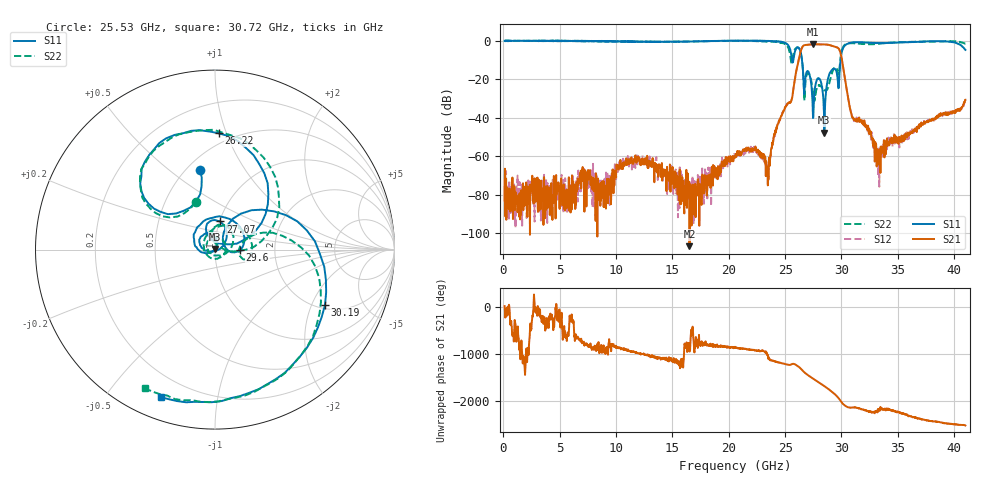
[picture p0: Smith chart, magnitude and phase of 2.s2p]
!The following data was pulled from an Agilent PNA
!This sNp file was generated from the data in the RF Test software
!NOTE:  Smoothing/Math/Corrections applied on any given trace ARE included in the data saved here
# MHz S dB R 50
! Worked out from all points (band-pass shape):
!   1601 points, 100 MHz to 41 GHz, reference 50 ohm
!   highest |S21| = -1.73 dB at 27.48 GHz (marker M1); lowest = -106.6 dB at 16.51 GHz (marker M2)
!   |S21| within 3 dB of the highest: 26.42 GHz to 29.82 GHz (3.401 GHz wide, 12.1 % of centre)
!   lowest |S11| = -47.7 dB at 28.47 GHz (marker M3), VSWR 1.01, Z = 50 + j0.411 ohm
!   |S11| at or under -10 dB: 25.61358 GHz to 25.72955 GHz (116 MHz wide, 0.452 % of centre); 26.5 GHz to 29.92 GHz (3.42 GHz wide, 12.1 % of centre)
!   |S22| runs from -31.2 to 0.2 dB; largest |S21 - S12| = 0.0062
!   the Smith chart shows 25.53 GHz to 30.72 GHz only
!   S11 on the Smith chart (normalised r, x): 25.53 GHz: 0.58, +0.65; 26.22 GHz: 0.42, +0.94; 27.07 GHz: 1.01, +0.32; 29.6 GHz: 1.32, -0.00; 30.19 GHz: 2.17, -2.52; 30.72 GHz: 0.10, -0.70
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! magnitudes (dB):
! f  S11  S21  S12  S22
! 100 MHz  0.0  -82.9  -75.6  0.0
! 6.925 GHz  -0.1  -68.3  -71.2  -0.2
! 8.536 GHz  -0.3  -76.6  -79.5  -0.2
! 10.99 GHz  -0.3  -62.7  -62.0  -0.5
! 13.75 GHz  -0.5  -66.3  -67.1  -0.5
! 16.51 GHz  -0.4  -106.6  -77.9  -0.4
! 20.55 GHz  0.1  -60.2  -60.6  -0.1
! 23.46 GHz  -0.1  -75.0  -69.6  -0.4
! 25.53 GHz  -7.0  -31.2  -31.4  -10.9
! 26.22 GHz  -3.8  -9.1  -9.0  -3.9
! 27.07 GHz  -15.9  -2.0  -2.0  -16.9
! 27.38 GHz  -26.1  -1.8  -1.8  -22.6
! 27.48 GHz  -40.1  -1.7  -1.8  -27.1
! 27.99 GHz  -19.7  -1.9  -1.9  -23.3
! 28.47 GHz  -47.7  -1.9  -1.9  -25.6
! 29.04 GHz  -16.0  -2.4  -2.4  -19.3
! 29.6 GHz  -17.1  -3.4  -3.4  -14.5
! 30.19 GHz  -3.3  -15.0  -15.1  -2.8
! 30.72 GHz  -1.2  -34.1  -33.7  -1.3
! 33.25 GHz  -1.2  -57.3  -70.4  -1.6
! 34.2 GHz  -1.1  -52.3  -50.9  -1.1
! 41 GHz  -4.7  -30.6  -30.4  -1.5
